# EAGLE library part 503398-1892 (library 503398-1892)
MicroSD SMT Push-Push 1.28mm height MicroSD SMT Push-Push 1.28mm height Source: Datasheet
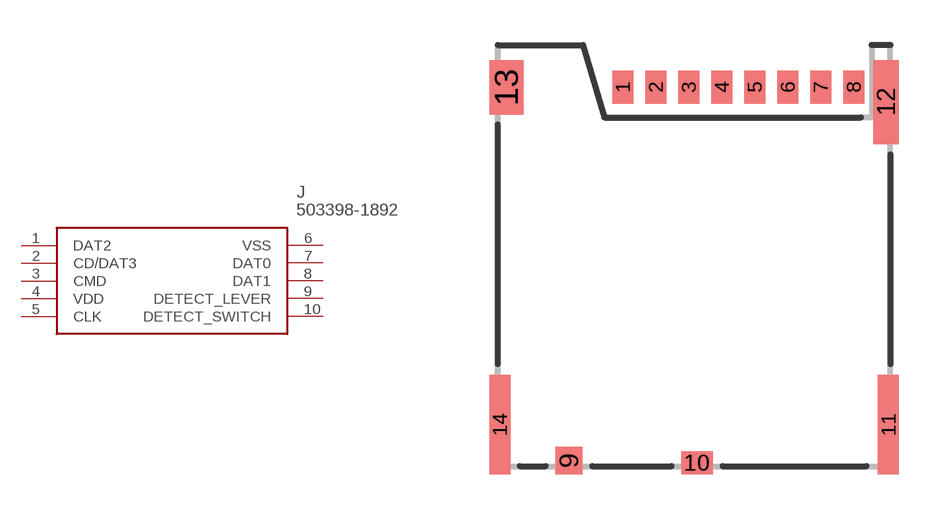
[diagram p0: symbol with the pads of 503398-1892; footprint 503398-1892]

Designator prefix J

## 503398-1892 (Description: MicroSD SMT Push-Push 1.28mm height MicroSD SMT Push-Push 1.28mm height; Height: mm; Manufacturer_Name: Molex; Manufacturer_Part_Number: 503398-1892; Mouser_Part_Number: 538-503398-1892; Mouser_Price-Stock: https://www.mouser.co.uk/ProductDetail/Molex/503398-1892?qs=b0v8CoHHvSMxV%252BW12iKaSg%3D%3D)  [503398-1892]
1  DAT2
2  CD/DAT3
3  CMD
4  VDD
5  CLK
6  VSS
7  DAT0
8  DAT1
9  DETECT_LEVER
10  DETECT_SWITCH

## Footprint 503398-1892 (pad centres in mm)
503398-1892
smd 0.7 x 1.1: 1 4.17,-1.4; 2 5.27,-1.4; 3 6.37,-1.4; 4 7.47,-1.4; 5 8.57,-1.4; 6 9.67,-1.4; 7 10.77,-1.4; 8 11.87,-1.4
smd 0.9 x 0.93: 9 2.38,-13.865
smd 1.05 x 0.78: 10 6.645,-13.94
smd 0.7 x 3.33: 11 13.03,-12.665; 14 0.07,-12.665
smd 0.86 x 2.8: 12 12.95,-1.9
smd 1.14 x 1.83: 13 0.29,-1.415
